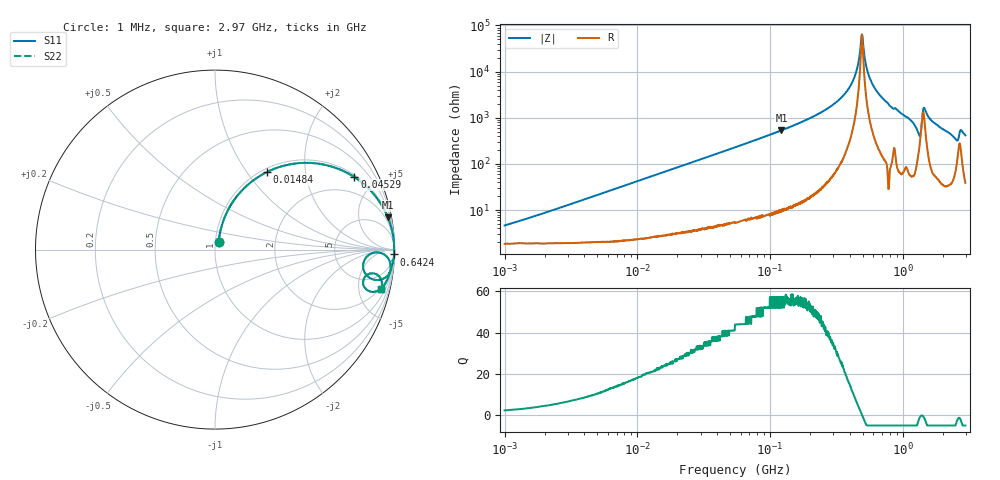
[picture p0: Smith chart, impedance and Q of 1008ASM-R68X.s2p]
!s-Parameter Generated by FASTRON Sdn. Bhd.
!FASTRON P/N : 1008ASM-R68X
!Keysight Technologies: E4991B_MY54100416_A.01.15
!Date: Tue Nov 21 09:30:00 2023
!Version  :Rev00  Wed Nov 22 15:16:59 2023
!Data & Calibration Information:
!Freq  S11  S21  S12  S22
!PortZ  Port1:50+j0  Port2:50+j0
!When reading reference impedance value at option line is always used.
! Remarks : This data is being provided solely for informational purposes.
# Hz S dB R 50
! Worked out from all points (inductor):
!   1599 points, 1 MHz to 2.97 GHz, reference 50 ohm
!   read as one part in series: L = 677 nH near 1.357 MHz
!   highest Q = 57.2 at 122 MHz (marker M1), where L = 694 nH
!   self-resonance near 492.7 MHz
!   S11 on the Smith chart (normalised r, x): 1 MHz: 1.04, +0.09; 14.84 MHz: 1.05, +1.25; 45.29 MHz: 1.09, +3.79; 642.4 MHz: 6, -73; 2.97 GHz: 1.78, -8.26
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1000000  -26.80 64.1  -0.17 -2.4  -0.17 -2.4  -26.80 64.1
3804036  -16.10 74.0  -0.28 -9.0  -0.28 -9.0  -16.10 74.0
1.439846e7  -5.87 56.9  -1.53 -30.6  -1.53 -30.6  -5.87 56.9
1.483731e7  -5.68 56.2  -1.60 -31.3  -1.60 -31.3  -5.68 56.2
4.528757e7  -1.15 27.5  -6.72 -61.1  -6.72 -61.1  -1.15 27.5
5.477226e7  -0.83 23.3  -8.06 -65.4  -8.06 -65.4  -0.83 23.3
1.219755e8  -0.18 10.6  -14.70 -78.4  -14.70 -78.4  -0.18 10.6
2.073156e8  -0.06 5.5  -20.30 -83.3  -20.30 -83.3  -0.06 5.5
3.017325e8  -0.02 2.9  -25.90 -85.4  -25.90 -85.4  -0.02 2.9
3.894533e8  -0.02 1.4  -32.40 -85.1  -32.40 -85.1  -0.02 1.4
4.435663e8  -0.01 0.6  -39.30 -81.5  -39.30 -81.5  -0.01 0.6
4.92715e8  -0.01 0.0  -56.10 -6.0  -56.10 -6.0  -0.01 0.0
5.528145e8  -0.01 -0.7  -38.70 81.2  -38.70 81.2  -0.01 -0.7
6.423554e8  -0.02 -1.6  -31.30 84.5  -31.30 84.5  -0.02 -1.6
7.846996e8  -0.02 -3.0  -25.80 86.2  -25.80 86.2  -0.02 -3.0
1.130699e9  -0.11 -6.1  -19.40 80.3  -19.40 80.3  -0.11 -6.1
1.320433e9  -0.89 -10.7  -13.90 56.2  -13.90 56.2  -0.89 -10.7
1.466741e9  -0.28 -3.1  -24.10 58.5  -24.10 58.5  -0.28 -3.1
1.67892e9  -0.14 -6.8  -18.50 78.8  -18.50 78.8  -0.14 -6.8
2.480502e9  -0.69 -14.7  -11.80 65.5  -11.80 65.5  -0.69 -14.7
2.75535e9  -0.64 -9.3  -15.30 61.0  -15.30 61.0  -0.64 -9.3
2.970126e9  -0.43 -13.2  -12.80 71.4  -12.80 71.4  -0.43 -13.2
